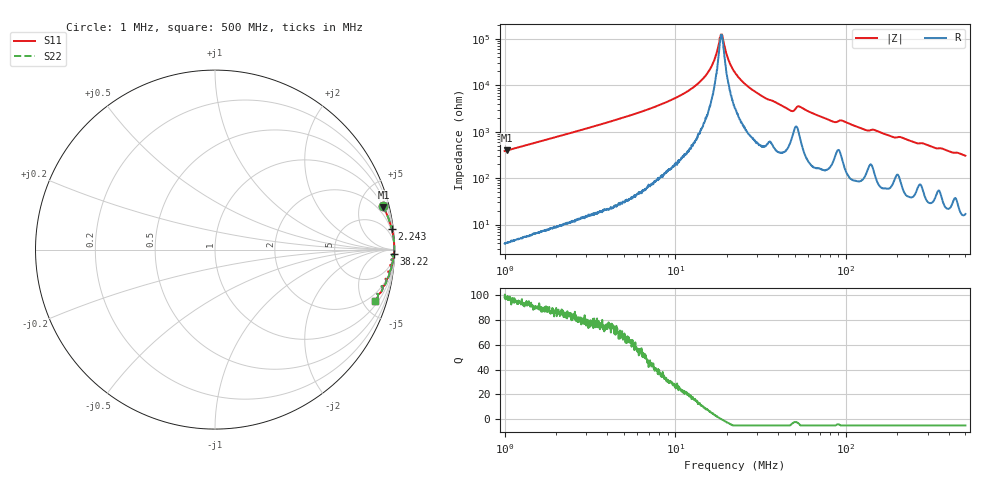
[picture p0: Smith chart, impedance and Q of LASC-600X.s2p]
!s-Parameter Generated by FASTRON Sdn. Bhd.
!FASTRON P/N : LASC-600X
!Keysight Technologies,E4991B,MY54100416,A.01.15
!Date: Tue Mar 17 14:45:35 2026
!Version  : Rev00 Tue Mar 17 14:45:35 2026
!Data & Calibration Information:
!PortZ  Port1:50+j0  Port2:50+j0
!When reading, reference impedance value at option line is always used.
!Remarks : This data is being provided solely for informational purposes.
!Freq	S11	S21	S12	S22
# Hz S dB R 50
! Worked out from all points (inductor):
!   1601 points, 1 MHz to 500 MHz, reference 50 ohm
!   read as one part in series: L = 60.9 uH near 1.032 MHz
!   highest Q = 98 at 1.036 MHz (marker M1), where L = 61.1 uH
!   self-resonance near 18.56 MHz
!   S11 on the Smith chart (normalised r, x): 1 MHz: 1.08, +7.68; 2.243 MHz: 1, +17; 38.22 MHz: 10, -88; 500 MHz: 1.34, -6.09
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1000000  -0.31 14.6  -12.00 -74.9  -12.00 -74.9  -0.31 14.6
1035575  -0.29 14.1  -12.28 -75.3  -12.28 -75.3  -0.29 14.1
2243190  -0.07 6.6  -18.84 -82.7  -18.84 -82.7  -0.07 6.6
2820919  -0.05 5.2  -20.87 -84.1  -20.87 -84.1  -0.05 5.2
7957584  -0.01 1.5  -31.37 -87.0  -31.37 -87.0  -0.01 1.5
1.155366e7  -0.01 0.8  -37.07 -86.5  -37.07 -86.5  -0.01 0.8
1.447295e7  -0.01 0.4  -42.77 -84.2  -42.77 -84.2  -0.01 0.4
1.65162e7  -0.01 0.2  -49.17 -77.7  -49.17 -77.7  -0.01 0.2
1.855735e7  -0.01 0.0  -61.56 -9.4  -61.56 -9.4  -0.01 0.0
1.906882e7  -0.01 -0.0  -59.65 36.4  -59.65 36.4  -0.01 -0.0
2.06894e7  -0.01 -0.2  -50.24 73.3  -50.24 73.3  -0.01 -0.2
2.236068e7  -0.01 -0.3  -45.48 79.8  -45.48 79.8  -0.01 -0.3
2.768612e7  -0.01 -0.7  -38.58 84.0  -38.58 84.0  -0.01 -0.7
3.821828e7  -0.02 -1.3  -32.93 83.1  -32.93 83.1  -0.02 -1.3
4.750454e7  -0.07 -1.9  -29.15 75.2  -29.15 75.2  -0.07 -1.9
5.316844e7  -0.06 -1.6  -30.98 74.1  -30.98 74.1  -0.06 -1.6
6.307767e7  -0.03 -2.2  -28.11 83.6  -28.11 83.6  -0.03 -2.2
8.408199e7  -0.09 -3.4  -24.44 78.6  -24.44 78.6  -0.09 -3.4
9.484087e7  -0.09 -3.2  -24.91 78.4  -24.91 78.4  -0.09 -3.2
1.294029e8  -0.11 -5.1  -20.96 79.0  -20.96 79.0  -0.11 -5.1
1.77937e8  -0.13 -6.8  -18.56 79.2  -18.56 79.2  -0.13 -6.8
5e8  -0.58 -17.8  -10.27 69.0  -10.27 69.0  -0.58 -17.8
